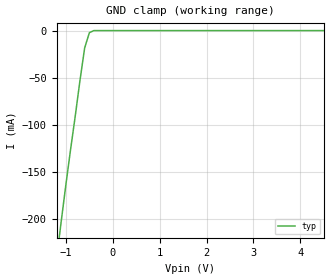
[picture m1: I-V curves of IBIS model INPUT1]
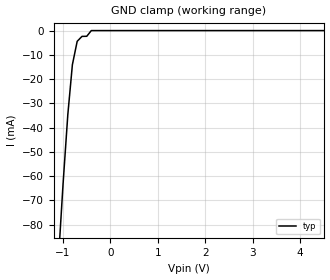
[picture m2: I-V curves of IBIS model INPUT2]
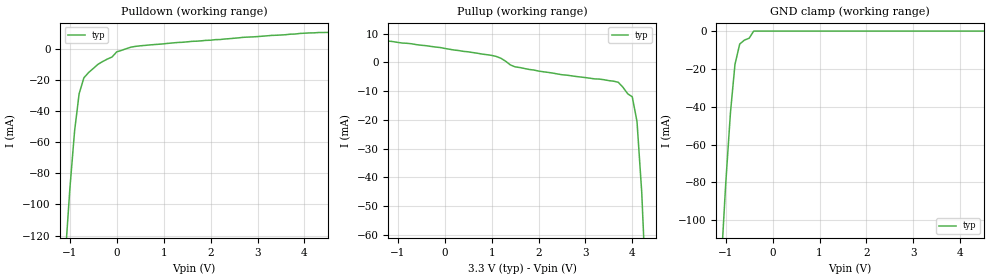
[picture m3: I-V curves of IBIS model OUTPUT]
|   PERICOM SEMICONDUCTOR CORP
|   IBIS Model of PI6C48543
|   Product Family: 6C
|   TSSOP Package (L)
[IBIS Ver] 3.2
[Comment char] |_char
[File Name] 6c48543.ibs
[File Rev] 2.0
[Source] File originated at Pericom Semiconductor Corp.
[Date] 10/13/2011
[Disclaimer] (C) Copyright PERICOM Semiconductor Corporation
   All rights reserved
  Pericom Semiconductor Corporation hereby grants the user of
  this IBIS model a non-exclusive, nontransferable license to
  use this IBIS model under the following terms.
  This IBIS model is provided on an "AS IS" basis and Pericom
  makes absolutely no warranty with respect to the information
  contained herein. PERICOM DISCLAIMS AND CUSTOMER WAIVES ALL
  WARRANTIES, EXPRESSED OR IMPLIED, INCLUDING WARRANTIES OF
  MERCHANTABILITY OR FITNESS FOR A PARTICULAR PURPOSE. The
  entire risk as to quality and performance is with the customer.
  Accordingly, in no event shall the company be liable for any
  damages, whether in contract or tort, including any lost
  profits or other incidental, consequential, exemplary, or
  punitive damages arising out of the use or application of the
  IBIS model provided in this package. Further, Pericom reserves
  the right to make changes without notice to any product herein
  to improve reliability, function, or design. Pericom does not
  convey any license under patent rights or any other intellectual
  property rights, including those of third parties.
  The user is granted this license only to use the IBIS model
  and is not granted rights to sell, load, rent, lease or license
  the IBIS model in whole or in part, or in modified form to anyone
  other than user. User may modify the IBIS model to suit its specific
  application but rights to derivative works and such modifications
  shall belong to Pericom.
  Pericom is not obligated to provide maintenance or support
  for the licensed IBIS model.
  Contact Pericom at ATTN: APPLICATIONS ENGINEERING / IBIS MODELS
  3545 North first street, San Jose, CA 95134
[Component] PI6C48543
[Manufacturer] Pericom Semiconductor Corp.
[Package]
| variable   typ   min  max
R_pkg   0.03869ohm   NA   NA
L_pkg   2.64482nH   NA   NA
C_pkg   0.19279pF   NA   NA
[Pin]   signal_name   model_name   R_pin   L_pin   C_pin
1   GND   GND   0.04069   3.22001nH   0.23014pF
2   CLK_EN   INPUT1   0.03969   2.93241nH   0.21146pF
3   CLK_SEL   INPUT1   0.03869   2.64482nH   0.19279pF
4   CLK   INPUT2   0.03768   2.35722nH   0.17411pF
5   nCLK   INPUT2   0.03768   2.35722nH   0.17411pF
6   PCLK   INPUT2   0.03768   2.35722nH   0.17411pF
7   nPCLK   INPUT2   0.03768   2.35722nH   0.17411pF
8   OE   INPUT1   0.03869   2.64482nH   0.19279pF
9   GND   GND   0.03969   2.93241nH   0.21146pF
10   VCC   POWER   0.04069   3.22001nH   0.23014pF
11   nQ3   OUTPUT   0.04069   3.22001nH   0.23014pF
12   Q3   OUTPUT   0.03969   2.93241nH   0.21146pF
13   GND   GND   0.03869   2.64482nH   0.19279pF
14   nQ2   OUTPUT   0.03768   2.35722nH   0.17411pF
15   Q2   OUTPUT   0.03668   2.06962nH   0.15543pF
16   nQ1   OUTPUT   0.03668   2.06962nH   0.15543pF
17   Q1   OUTPUT   0.03768   2.35722nH   0.17411pF
18   VCC   POWER   0.03869   2.64482nH   0.19279pF
19   nQ0   OUTPUT   0.03969   2.93241nH   0.21146pF
20   Q0   OUTPUT   0.04069   3.22001nH   0.23014pF
[Diff Pin]  inv_pin vdiff   tdelay_typ tdelay_min tdelay_max
12   11   NA   NA   NA   NA
15   14   NA   NA   NA   NA
17   16   NA   NA   NA   NA
20   19   NA   NA   NA   NA
| Models and submodels in the file (3): INPUT1 (Input), INPUT2 (Input), OUTPUT (Output)
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|   Model INPUT1
[Model] INPUT1
Model_type Input
Vinl =  0.800V
Vinh =  2.000V
| variable   typ   min   max
C_comp   6.000pF   NA   NA
[Voltage Range]   3.300V   NA   NA
[GND Clamp Reference]   0.000V   NA   NA
[POWER Clamp Reference]   3.300V   NA   NA
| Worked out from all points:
|   GND clamp passes 1 mA (typ) near -0.45 V on its own axis
[GND Clamp]
| Voltage   I(typ)   I(min)  I(max)
-3.3V     -1.193A    NA         NA
-1.202V   -243.8mA   NA         NA
-1.101V   -202.6mA   NA         NA
-999.5mV  -163.1mA   NA         NA
-898.4mV  -125.5mA   NA         NA
-802.2mV  -91.25mA   NA         NA
-701mV    -53.26mA   NA         NA
-599.9mV  -18.38mA   NA         NA
-498.8mV  -2.21mA    NA         NA
-402.9mV  0A         NA         NA
6.601V    0A         NA         NA
[POWER Clamp]   |Note: Vtable = Vcc - Voutput
| Voltage   I(typ)   I(min)   I(max)
-3.3V     0A         NA         NA
0V        0A         NA         NA
|   Model INPUT2
[Model] INPUT2
Model_type Input
Vinl =  1.300V
Vinh =  2.000V
| variable   typ   min   max
C_comp   6.000pF   NA   NA
[Voltage Range]   3.300V   NA   NA
[GND Clamp Reference]   0.000V   NA   NA
[POWER Clamp Reference]   3.300V   NA   NA
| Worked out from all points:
|   GND clamp passes 1 mA (typ) near -0.44 V on its own axis
[GND Clamp]
| Voltage   I(typ)   I(min)  I(max)
-3.3V     -833.8mA   NA         NA
-1.101V   -95.76mA   NA         NA
-999.5mV  -63.43mA   NA         NA
-898.4mV  -34.62mA   NA         NA
-802.2mV  -14.09mA   NA         NA
-701mV    -4.43mA    NA         NA
-599.9mV  -2.4mA     NA         NA
-498.8mV  -2.35mA    NA         NA
-402.9mV  0A         NA         NA
6.602V    0A         NA         NA
[POWER Clamp]   |Note: Vtable = Vcc - Voutput
| Voltage   I(typ)   I(min)   I(max)
-3.3V     0A         NA         NA
0V        0A         NA         NA
|   Model OUTPUT
[Model]   OUTPUT
Model_type  Output
Vref =  1.20V
Vmeas = 1.20V
| variable   typ   min   max
C_comp   10.000pF  NA   NA
[Voltage Range]   3.300V   NA   NA
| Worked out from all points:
|   slope of the pulldown table from 0 to 0.495 V, typ, clamps not added: 128 ohm
|   slope of the pullup table from 0 to 0.495 V, typ, clamps not added: 420 ohm
|   GND clamp passes 1 mA (typ) near -0.43 V on its own axis
[GND Clamp]
| Voltage   I(typ)   I(min)  I(max)
-3.301V   -979.2mA   NA         NA
-1.1V     -125.3mA   NA         NA
-999.3mV  -80.9mA    NA         NA
-898.1mV  -43.12mA   NA         NA
-802mV    -17.66mA   NA         NA
-700.8mV  -6.86mA    NA         NA
-599.6mV  -4.75mA    NA         NA
-498.4mV  -3.75mA    NA         NA
-402.7mV  0A         NA         NA
6.6V      0A         NA         NA
[Pulldown]
| Voltage   I(typ)   I(min)  I(max)
-3.3V     -1.224A    NA         NA
-1.1V     -134.8mA   NA         NA
-999.3mV  -89.86mA   NA         NA
-898.2mV  -52.71mA   NA         NA
-802mV    -28.96mA   NA         NA
-700.8mV  -18.74mA   NA         NA
-599.7mV  -15.33mA   NA         NA
-1.89mV   -2.1mA     NA         NA
498.4mV   1.8mA      NA         NA
2.698V    7.25mA     NA         NA
4.301V    10.33mA    NA         NA
6.6V      11.69mA    NA         NA
[Pullup]   |Note: Vtable = Vcc - Voutput
| Voltage   I(typ)   I(min)  I(max)
-3.3V     11.36mA    NA         NA
-700.7mV  6.5mA      NA         NA
999.1mV   2.48mA     NA         NA
1.202V    1.44mA     NA         NA
1.499V    -1.52mA    NA         NA
3.699V    -6.9mA     NA         NA
3.901V    -10.92mA   NA         NA
3.997V    -11.95mA   NA         NA
4.098V    -20.51mA   NA         NA
4.199V    -45.22mA   NA         NA
4.301V    -83.28mA   NA         NA
6.6V      -1.135A    NA         NA
[Ramp]
| variable   typ   min   max
dV/dt_r   0.18/142p   NA   NA
dV/dt_f   0.18/159p   NA   NA
R_load = 50ohms
